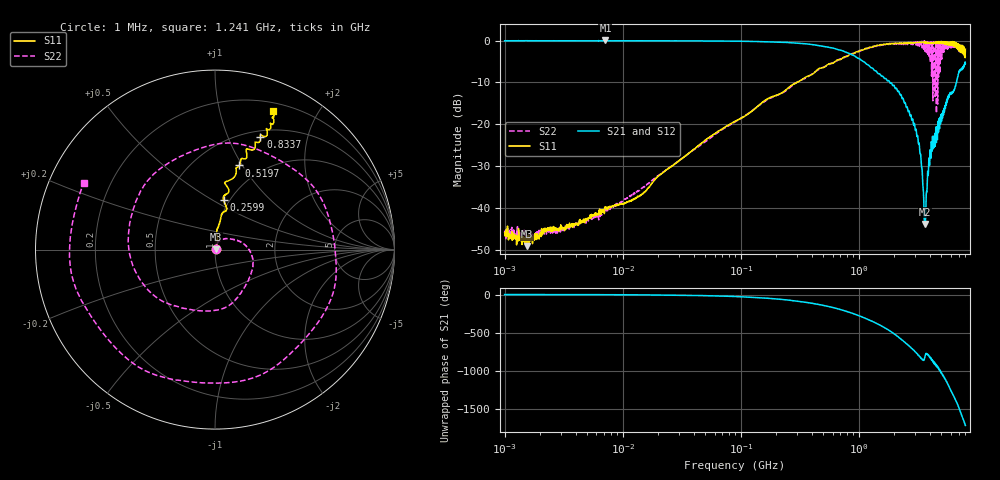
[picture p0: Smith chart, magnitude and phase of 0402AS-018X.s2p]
!s-Parameter Generated by FASTRON Sdn. Bhd.
!FASTRON P/N : 0402AS-018X
!Keysight Technologies: E5071C_MY46733604_B.14.02
!Date: Mon Dec 01 10:31:49 2025
!Version  :Rev00  Mon Dec 01 10:31:49 2025
!Data & Calibration Information:
!Freq  S11:SOLT2(ON)  S21:SOLT2(ON)  S12:SOLT2(ON)  S22:SOLT2(ON)
!PortZ  Port1:50+j0  Port2:50+j0
!When reading reference impedance value at option line is always used.
! Remarks : This data is being provided solely for informational purposes.
# Hz S dB R 50
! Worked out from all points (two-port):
!   1601 points, 1 MHz to 8 GHz, reference 50 ohm
!   highest |S21| = 0.03 dB at 7.138 MHz (marker M1); lowest = -43.9 dB at 3.609 GHz (marker M2)
!   |S21| within 3 dB of the highest: start of sweep to 813.8 MHz
!   lowest |S11| = -49.2 dB at 1.541 MHz (marker M3), VSWR 1.01, Z = 50.3 + j0.18 ohm
!   |S11| at or under -10 dB: start of sweep to 300.2 MHz
!   |S22| runs from -47.8 to -0.1 dB; largest |S21 - S12| = 0.023
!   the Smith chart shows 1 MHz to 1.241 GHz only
!   S11 on the Smith chart (normalised r, x): 1 MHz: 1.01, +0.00; 259.9 MHz: 0.94, +0.56; 519.7 MHz: 0.79, +0.97; 833.7 MHz: 0.57, +1.32; 1.241 GHz: 0.29, +1.46
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1000000  -45.90 23.0  -0.05 -0.3  -0.03 -0.3  -45.70 16.7
1541011  -49.20 31.1  -0.04 -0.5  -0.03 -0.5  -46.70 6.8
4479405  -43.40 51.7  -0.05 -1.4  -0.04 -1.4  -43.20 53.3
7138274  -39.90 54.6  0.03 -2.4  -0.05 -2.5  -40.20 57.4
2.00676e7  -32.40 69.9  -0.06 -6.0  -0.06 -5.9  -32.30 70.8
8.994653e7  -19.30 84.5  -0.14 -26.4  -0.14 -26.3  -19.40 33.3
2.598545e8  -11.10 80.2  -0.50 -75.0  -0.49 -75.0  -11.30 -55.0
4.006501e8  -8.13 78.7  -0.94 -115.0  -0.93 -115.0  -7.99 -131.0
5.196823e8  -6.23 73.9  -1.44 -148.0  -1.43 -148.0  -6.19 169.0
8.33667e8  -3.38 68.1  -3.11 126.0  -3.10 126.0  -3.55 3.8
1.035959e9  -2.30 66.3  -4.54 73.3  -4.54 73.1  -2.49 -102.0
1.241273e9  -1.56 67.3  -6.24 21.7  -6.25 21.5  -1.71 153.0
1.550632e9  -1.01 72.6  -8.47 -50.7  -8.48 -50.8  -0.99 3.1
1.7949e9  -0.78 77.6  -9.59 -108.0  -9.61 -108.0  -0.94 -116.0
2.093169e9  -0.64 83.4  -11.50 179.0  -11.50 179.0  -0.89 92.8
2.266813e9  -0.74 84.6  -12.90 139.0  -12.90 139.0  -0.77 10.9
2.457552e9  -0.72 87.8  -14.80 94.3  -14.80 94.3  -0.69 -82.0
2.824359e9  -0.61 96.4  -19.10 11.9  -19.10 11.8  -0.36 101.0
3.183204e9  -0.42 105.0  -24.00 -74.7  -23.90 -75.0  -0.80 -88.7
3.60885e9  -0.67 115.0  -43.90 -113.0  -44.00 -112.0  -0.05 76.5
3.912882e9  -0.68 121.0  -29.20 -75.6  -29.20 -76.1  -0.40 -65.8
8e9  -2.06 -117.0  -5.49 83.3  -5.51 82.9  -3.65 121.0
